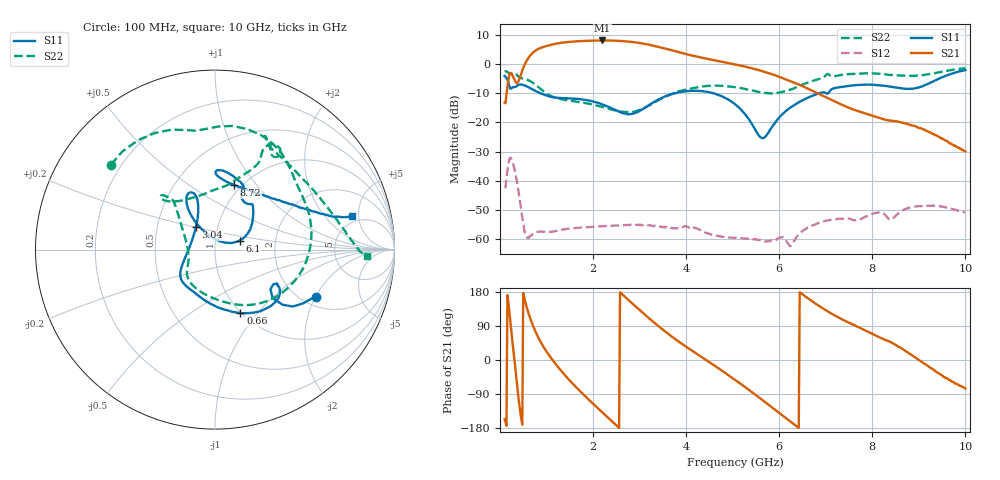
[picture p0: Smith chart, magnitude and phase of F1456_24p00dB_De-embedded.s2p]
! Integrated Device Technology
! Corporate Headquarters
! 6024 Silver Creek Valley Road
! San Jose, CA 95138  USA
! Phone:  1-408-284-8200
! Toll Free:  1-800-223-1366
! Webpage:  http://www.idt.com/
! Timing and RF Division
! 515 Groton Road, Suite 102
! Westford, MA 01886-6024
! Device:  F1456
! Description: 6-bit 0.5 dB Transmit Variable Gain Amplifier
! Frequency:  2100.0 -  2950.00 MHz
! Package:  6x6 mm Thin QFN Plastic Package: 28 pin
! State:  48
! Atten State:  24.0 dB
! Voltage:  +5.00 Volts
! Current:  216.974 mA
! Data:  The device was measured on a the F1455 evaluation board which has
!  individual transmission lines to the RF pins.  Data was collected
!  using a calibrated network analyzer.  The evaluation board was
!  de-embedded using a TRL calibration technique.
!  The reference plane is the edge of the package pin.
!  Pin  1 = CSb
!  Pin  2 = DATA
!  Pin  3 = CLK
!  Pin  4 = RSET
!  Pin  5 = GND
!  Pin  6 = RFIN  = Port 1
!  Pin  7 = GND
!  Pin  8 = NC
!  Pin  9 = NC
!  Pin 10 = NC
!  Pin 11 = NC
!  Pin 12 = NC
!  Pin 13 = NC
!  Pin 14 = /STBY
!  Pin 15 = GND
!  Pin 16 = RFOUT  = Port 2
!  Pin 17 = GND
!  Pin 18 = NC
!  Pin 19 = NC
!  Pin 20 = NC
!  Pin 21 = GND
!  Pin 22 = NC
!  Pin 23 = GND
!  Pin 24 = NC
!  Pin 25 = NC
!  Pin 26 = NC
!  Pin 27 = GND
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# GHz S dB R 50
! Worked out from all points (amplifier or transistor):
!   496 points, 100 MHz to 10 GHz, reference 50 ohm
!   highest |S21| = 8.0 dB at 2.2 GHz (marker M1)
!   |S21| within 3 dB of that: 813.3 MHz to 3.607 GHz (2.794 GHz wide, 126 % of centre)
!   unconditionally stable (mu >= 1): start of sweep to end of sweep
!   at 1.74 GHz: K = 114.25, MAG = 8.3 dB, |S12| = -56.0 dB
!   at 5.06 GHz: K = 388.74, MAG = 0.8 dB, |S12| = -59.5 dB
!   at 10 GHz: K = 594.42, MAG = -20.3 dB, |S12| = -50.8 dB
!   S11 on the Smith chart (normalised r, x): 100 MHz: 2.37, -2.02; 660 MHz: 0.99, -0.82; 3.04 GHz: 0.78, +0.20; 6.1 GHz: 1.31, +0.13; 8.72 GHz: 0.93, +0.78; 10 GHz: 4.18, +4.10
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0.1  -4.13 -24.9  -13.22 -156.5  -42.30 49.9  -2.52 140.8
0.24  -8.46 -30.9  -3.08 80.1  -32.28 -76.6  -3.42 94.5
0.32  -7.90 -29.7  -5.70 -9.1  -36.51 -154.3  -3.26 67.8
0.42  -7.05 -36.9  -5.05 -122.6  -45.80 140.0  -4.60 40.8
0.54  -7.41 -53.7  0.05 155.2  -58.07 130.2  -5.14 15.6
0.66  -8.40 -68.1  3.08 106.6  -58.83 145.4  -5.98 -11.7
0.84  -9.81 -86.8  5.26 55.5  -57.42 116.8  -8.09 -48.8
1.16  -11.41 -113.1  6.79 -4.9  -57.34 79.0  -11.39 -92.8
1.48  -11.77 -130.3  7.55 -51.5  -56.40 56.5  -12.51 -119.4
1.76  -12.12 -140.7  7.85 -87.0  -55.95 41.2  -13.16 -133.2
2.2  -13.82 -154.2  8.05 -138.3  -55.49 22.6  -14.71 -146.9
2.6  -16.59 -180.0  7.88 176.4  -55.25 6.7  -16.29 -163.3
3.04  -15.72 130.6  7.07 127.5  -55.10 -12.4  -15.48 163.6
3.4  -12.23 112.4  5.88 89.9  -55.58 -29.2  -12.48 142.7
4.1  -9.21 113.0  2.98 26.8  -56.27 -61.7  -8.43 131.2
5.06  -13.90 125.2  -0.17 -53.0  -59.52 -112.0  -7.95 136.2
5.64  -25.42 69.0  -2.48 -105.7  -60.57 -157.8  -9.81 120.5
6.1  -16.76 19.9  -5.02 -149.5  -59.63 165.9  -9.42 88.2
6.7  -10.97 41.3  -9.10 155.6  -55.34 147.7  -5.91 64.7
8.36  -7.69 88.2  -19.34 49.2  -53.23 66.7  -3.73 62.5
8.72  -8.52 73.4  -20.43 23.2  -49.56 69.4  -4.02 50.3
10  -2.10 13.8  -29.90 -75.1  -50.83 -23.7  -1.46 -2.6
